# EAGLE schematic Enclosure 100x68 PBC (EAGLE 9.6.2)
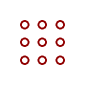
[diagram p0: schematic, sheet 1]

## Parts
U$1  PROTO-34X22-C  [PROTO-34X22-C]

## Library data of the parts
U$1 = digitalconcepts:PROTO-34X22-C: 34 x 22 Prototyping board, with cut-outs, to fit an 100 x 68 enclosure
